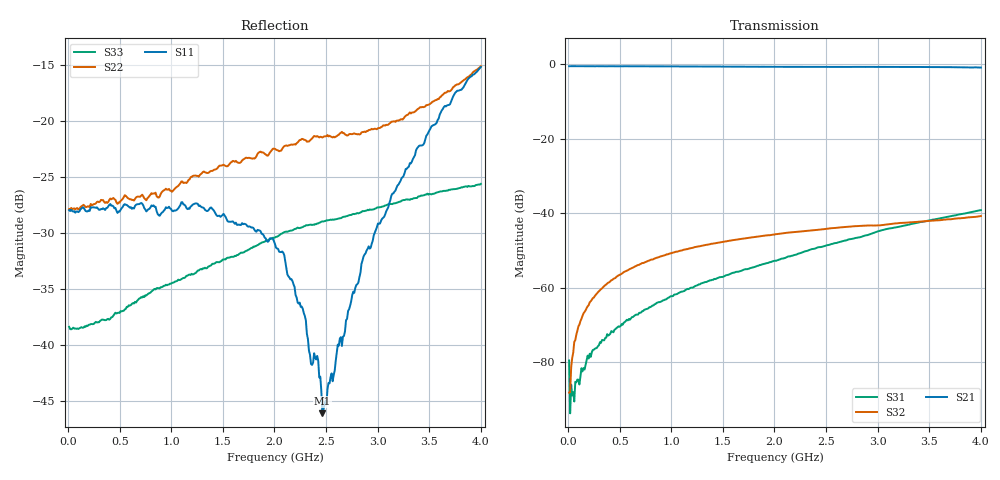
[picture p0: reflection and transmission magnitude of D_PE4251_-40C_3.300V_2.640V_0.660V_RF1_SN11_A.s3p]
! Device ID: PE4251_SoldCshunt_081809
! Dir: c:\Test Bench Repositories\Bench_Software_CVI_Version_8\trunk\PSC 4Port_VNA Bench\datalog\4250\TEST\PE4251_SoldCshunt_081809\-40C\3p300000\RF1
! Serial: 11
! Insertion: A
! Temp: -40C
! VDD: 3.300
! Control_Hi: 80.000
! Control_Lo: 20.000
! Logic State: RF1
! Port 1: RFC
! Port 2: RF1
! Port 3: RF2
! V1 = 0.66
! V2 = 2.64
! V3 = 0.66
! IDD: 5.000450e-05
! FILE NAME
! DATE 08/18/09  20:08
! CORRECTED  DATA
#  Hz  S  RI  R  50.00
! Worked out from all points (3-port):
!   401 points, 10 MHz to 4 GHz, reference 50 ohm
!   strongest paths, dB at 10 MHz, 1.008 GHz, 2.005 GHz, 3.002 GHz, 4 GHz:
!     S21: -0.5, -0.5, -0.6, -0.7, -0.9
!     S32: -88.2, -50.6, -45.7, -43.3, -40.7
!     S31: -79.5, -62.3, -52.7, -44.8, -39.2
!   lowest |S11| = -46.1 dB at 2.464 GHz (marker M1), VSWR 1.01, Z = 50.2 - j0.472 ohm
!   |S11| at or under -10 dB: start of sweep to end of sweep
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1e7  0.04 0.000185  0.9446 -0.00314  1.08e-05 -5.3e-05
     0.9447 -0.00411  0.0404 0.00028  5.27e-05 -1.52e-05
     0.000104 -1.59e-05  3.86e-05 5.95e-06  0.012 -0.000465
1.79575e8  0.0395 0.000819  0.9433 -0.061  -1.24e-05 -9.91e-05
           0.9427 -0.0608  0.0413 0.00059  4.33e-05 0.000535
           -8.95e-06 -0.000105  3.35e-05 0.000532  0.0121 0.00159
4.78825e8  0.0388 -0.00271  0.9296 -0.1594  -0.000136 -0.000254
           0.9285 -0.1594  0.0425 -0.00321  0.000135 0.00143
           -0.000145 -0.000256  0.000141 0.00143  0.0133 0.00382
1.02745e9  0.0374 -0.0136  0.8804 -0.3304  -0.000675 -0.000424
           0.8802 -0.3302  0.0478 -0.0129  0.000515 0.00294
           -0.000684 -0.000431  0.000509 0.00294  0.0161 0.0101
2.005e9  0.0263 -0.0101  0.7225 -0.5832  -0.00226 -0.000453
         0.7226 -0.5829  0.0664 -0.0351  0.00121 0.00506
         -0.00227 -0.000457  0.0012 0.00507  0.0186 0.0238
2.2843e9  0.0104 -0.00917  0.6671 -0.6432  -0.003 -0.000551
          0.6661 -0.6436  0.0646 -0.0514  0.00139 0.00559
          -0.003 -0.00056  0.00137 0.00559  0.017 0.0293
2.46385e9  0.00153 -0.0047  0.6303 -0.6781  -0.00351 -0.000495
           0.6289 -0.6776  0.0615 -0.0578  0.00137 0.00592
           -0.00352 -0.000525  0.00135 0.00595  0.0154 0.0321
2.86285e9  -0.0181 -0.017  0.538 -0.7547  -0.00493 -0.000441
           0.5384 -0.7524  0.0429 -0.0783  0.0015 0.00663
           -0.00494 -0.000438  0.0015 0.00664  0.0111 0.038
3.14215e9  -0.0363 -0.0303  0.4659 -0.7984  -0.00633 -2.86e-05
           0.4669 -0.798  0.0225 -0.0968  0.00116 0.00714
           -0.00633 -5.18e-05  0.00116 0.00714  0.00678 0.042
4e9  -0.1562 -0.0774  0.1855 -0.8891  -0.0108 0.00211
     0.1855 -0.8865  -0.1198 -0.1287  2.84e-05 0.00917
     -0.0108 0.00208  1.13e-05 0.00918  -0.0137 0.0505
